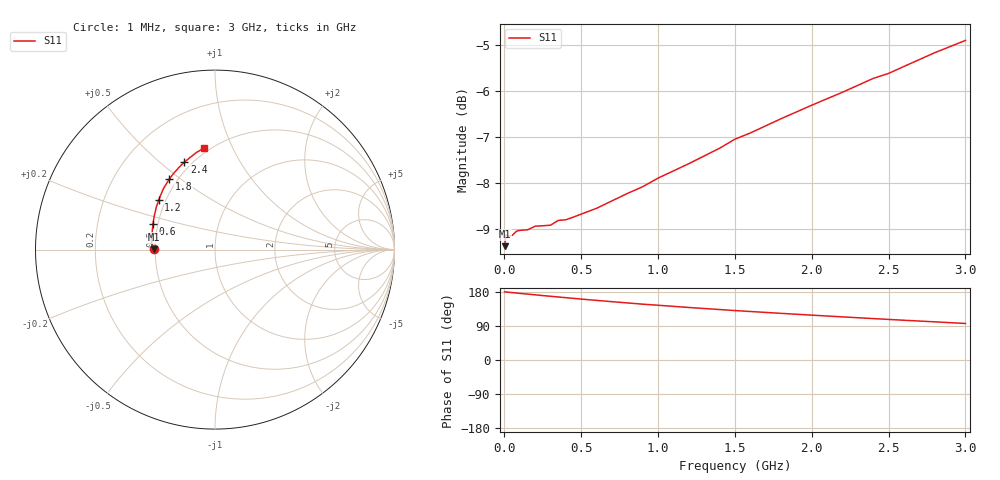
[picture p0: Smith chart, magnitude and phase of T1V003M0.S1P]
! SIEMENS Small Signal Semiconductors
! BAT68-04
! Si Schottky Diode (2 diodes in series, pin 3 open) in SOT23
! IF = 3 mA
! S-Parameters:  August  1994
# GHz  S  MA  R  50
!  f  S11
! GHz  MAG  ANG
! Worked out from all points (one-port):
!   33 points, 1 MHz to 3 GHz, reference 50 ohm
!   lowest |S11| = -9.4 dB at 1 MHz (marker M1), VSWR 2.03, Z = 24.6 + j0.033 ohm
!   |S11| at or under -10 dB: nowhere
!   S11 on the Smith chart (normalised r, x): 1 MHz: 0.49, +0.00; 600 MHz: 0.47, +0.16; 1.2 GHz: 0.46, +0.31; 1.8 GHz: 0.45, +0.45; 2.4 GHz: 0.46, +0.61; 3 GHz: 0.47, +0.78
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0.001  0.3399 179.9
0.01  0.3497 179.6
0.03  0.3484 178.6
0.05  0.3492 177.9
0.08  0.353 176.7
0.1  0.3536 175.8
0.15  0.3541 173.9
0.2  0.3573 172.0
0.3  0.3582 168.2
0.35  0.3625 166.3
0.4  0.3631 164.4
0.5  0.3683 160.7
0.6  0.3737 157.3
0.8  0.3878 150.6
0.9  0.3944 147.3
1  0.403 144.5
1.2  0.4178 138.6
1.4  0.4342 133.2
1.5  0.4442 130.5
1.6  0.4511 128.0
1.8  0.4675 123.1
2  0.4836 118.4
2.2  0.4995 113.8
2.4  0.5171 109.3
2.5  0.5236 107.1
2.6  0.5328 104.9
2.8  0.5514 100.7
3  0.5686 96.4
